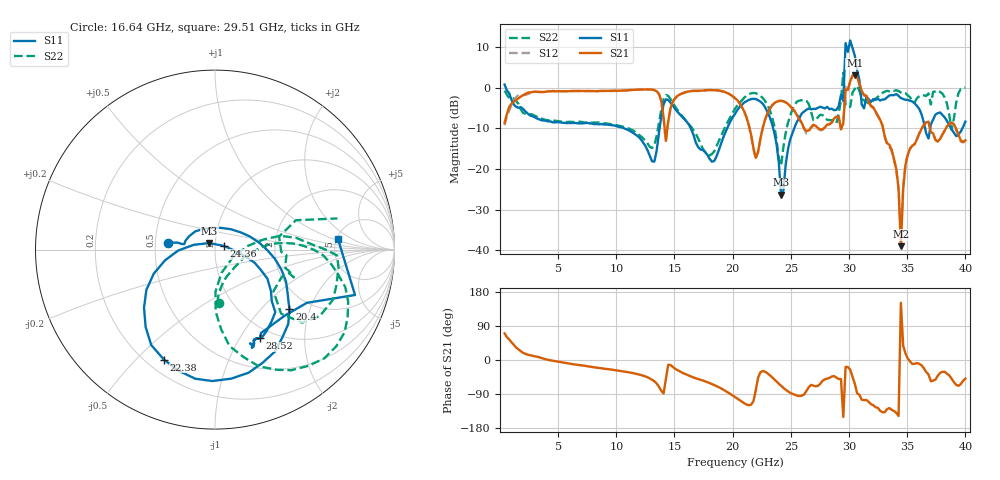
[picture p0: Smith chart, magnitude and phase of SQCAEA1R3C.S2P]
! Network Analyzer HP8722ES.07.66: Jul 25, 2000 Serial No. US39175408
! 26 Oct 2004  10:51:29
! Frequency  S11  S21  S12  S22
# HZ  S  DB R  50
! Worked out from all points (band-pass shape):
!   201 points, 400 MHz to 40 GHz, reference 50 ohm
!   highest |S21| = 3.04 dB at 30.5 GHz (marker M1); lowest = -39.0 dB at 34.46 GHz (marker M2)
!   |S21| within 3 dB of the highest: 29.95 GHz to 31 GHz (1.056 GHz wide, 3.46 % of centre)
!   lowest |S11| = -26.3 dB at 24.16 GHz (marker M3), VSWR 1.10, Z = 46.8 + j3.4 ohm
!   |S11| at or under -10 dB: 10.69 GHz to 13.72 GHz (3.027 GHz wide, 24.8 % of centre); 16.4 GHz to 19.52 GHz (3.116 GHz wide, 17.3 % of centre); 23.48 GHz to 25.29 GHz (1.805 GHz wide, 7.4 % of centre)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
!   |S22| runs from -19.2 to 3.7 dB; largest |S21 - S12| = 0.21
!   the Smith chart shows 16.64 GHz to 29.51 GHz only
!   S11 on the Smith chart (normalised r, x): 16.64 GHz: 0.59, +0.05; 20.4 GHz: 1.58, -1.47; 22.38 GHz: 0.27, -0.61; 24.36 GHz: 1.10, +0.05; 28.52 GHz: 0.86, -1.23; 29.51 GHz: 5.12, +1.17
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4e8  0.81 -20.9  -8.59 70.3  -9.23 75.5  -0.69 -12.5
7.132e9  -8.76 -115.6  -0.79 -14.6  -0.84 -15.4  -8.50 -95.8
1.3666e10  -11.09 19.3  -1.50 -70.7  -1.58 -71.9  -8.71 -14.1
1.6636e10  -11.59 171.6  -0.75 -46.0  -0.73 -46.2  -10.48 -86.1
2.02e10  -6.42 -31.9  -2.59 -98.1  -2.54 -98.9  -5.16 -0.1
2.0398e10  -5.49 -38.8  -3.01 -101.8  -3.16 -102.7  -4.38 -3.0
2.2378e10  -3.40 -114.9  -12.63 -32.4  -12.61 -32.1  -1.99 -57.8
2.416e10  -26.32 131.3  -3.19 -68.0  -3.18 -68.9  -19.18 -20.8
2.4358e10  -25.39 22.8  -3.32 -73.5  -3.31 -74.3  -14.60 6.6
2.6932e10  -5.19 -66.6  -9.12 -67.6  -9.16 -69.0  -7.97 -35.4
2.8516e10  -5.14 -63.0  -8.55 -43.5  -8.52 -45.0  -7.97 -4.5
2.9506e10  -3.25 5.0  -8.73 -150.3  -8.09 -132.7  3.71 33.5
2.9704e10  11.01 -5.0  -0.40 -18.0  0.45 -7.5  -4.29 -49.2
2.9902e10  8.84 -60.9  -0.44 -18.7  -0.58 -19.5  -4.78 16.4
3.01e10  11.66 -77.8  1.63 -25.4  1.57 -26.7  -4.68 23.5
3.0496e10  7.93 -107.5  3.04 -62.6  2.98 -63.4  -0.28 -5.6
3.0694e10  4.34 46.4  2.61 -87.9  2.44 -87.4  0.50 156.0
3.1486e10  -2.30 -101.6  -1.95 -105.4  -1.98 -108.2  -3.49 -24.8
3.3466e10  -1.88 -89.8  -14.03 -127.0  -14.51 -127.9  -0.85 -16.8
3.4456e10  -2.54 -103.5  -39.00 150.8  -36.17 131.6  -1.13 -24.4
3.6238e10  -6.57 -142.8  -10.05 -14.1  -10.06 -15.8  -1.76 -4.8
4e10  -8.32 -81.1  -12.92 -49.2  -13.02 -49.4  0.02 -11.0
